TYPE STR_EL1889 :
STRUCT
	In_Bit0		:	BOOL	;
	In_Bit1		:	BOOL	;
	In_Bit2		:	BOOL	;
	In_Bit3		:	BOOL	;
	In_Bit4		:	BOOL	;
	In_Bit5		:	BOOL	;
	In_Bit6		:	BOOL	;
	In_Bit7		:	BOOL	;
	In_Bit8		:	BOOL	;
	In_Bit9		:	BOOL	;
	In_Bit10		:	BOOL	;
	In_Bit11		:	BOOL	;
	In_Bit12		:	BOOL	;
	In_Bit13		:	BOOL	;
	In_Bit14		:	BOOL	;
	In_Bit15		:	BOOL	;

END_STRUCT
END_TYPE
